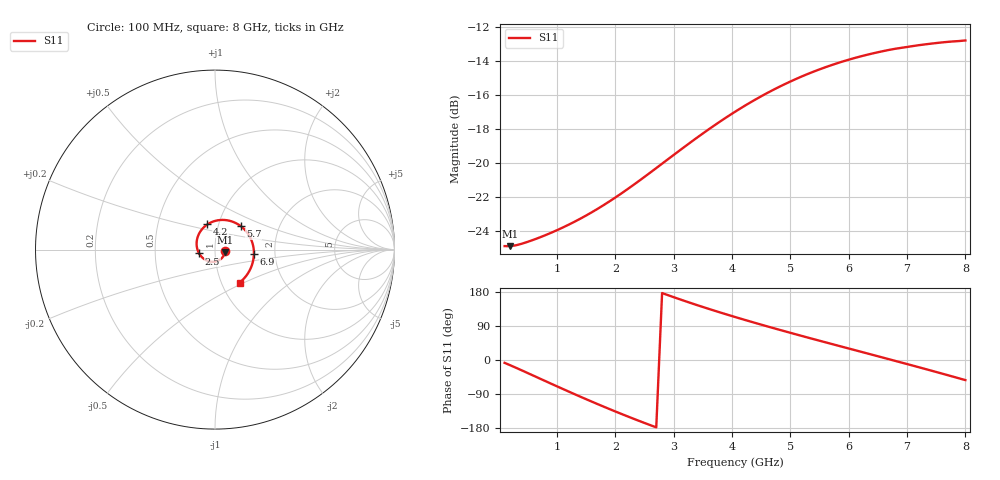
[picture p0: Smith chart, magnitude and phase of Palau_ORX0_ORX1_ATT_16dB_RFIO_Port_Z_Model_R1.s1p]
! Created Fri Oct  9 14:28:40 2020
! Palau ORX0/ORX1 RFIO Port Impedance Model.
! Attenuation  : 16 dB.
! Revision		: R1.
! Impedance Mode 	: Balanced Differential-Mode.
! Impedance Format 	: Series Equivalent Differential Impedance (SEDZ).
# hz S ma R 100
! 1 Port Network Data from SP1.SP block
! freq  magS11  angS11
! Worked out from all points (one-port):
!   80 points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, 100 MHz to 8 GHz, reference 100 ohm
!   lowest |S11| = -24.9 dB at 200 MHz (marker M1), VSWR 1.12, Z = 112 - j3.11 ohm
!   |S11| at or under -10 dB: start of sweep to end of sweep
!   S11 on the Smith chart (normalised r, x): 100 MHz: 1.12, -0.02; 2.5 GHz: 0.84, -0.04; 4.2 GHz: 0.88, +0.25; 5.7 GHz: 1.28, +0.35; 6.9 GHz: 1.55, -0.08; 8 GHz: 1.22, -0.47
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1e8  0.0569 -7.5
2e8  0.05688 -14.1
6e8  0.05944 -41.7
1.1e9  0.06458 -76.5
1.4e9  0.06856 -96.9
1.6e9  0.07166 -110.2
1.8e9  0.07518 -123.2
2.1e9  0.08128 -142.2
2.5e9  0.09104 -166.2
2.8e9  0.09949 176.7
3.1e9  0.1088 160.4
3.3e9  0.1154 150.0
3.6e9  0.1256 134.9
3.8e9  0.1326 125.2
4.1e9  0.1432 111.2
4.2e9  0.1467 106.7
4.5e9  0.1571 93.3
4.7e9  0.1639 84.5
5.1e9  0.1768 67.5
5.4e9  0.1858 55.0
5.7e9  0.1939 42.6
6.1e9  0.2036 26.3
6.5e9  0.2118 9.9
6.9e9  0.2182 -6.6
7.1e9  0.2208 -14.8
7.5e9  0.2254 -31.6
7.7e9  0.2272 -40.2
8e9  0.2294 -53.1
